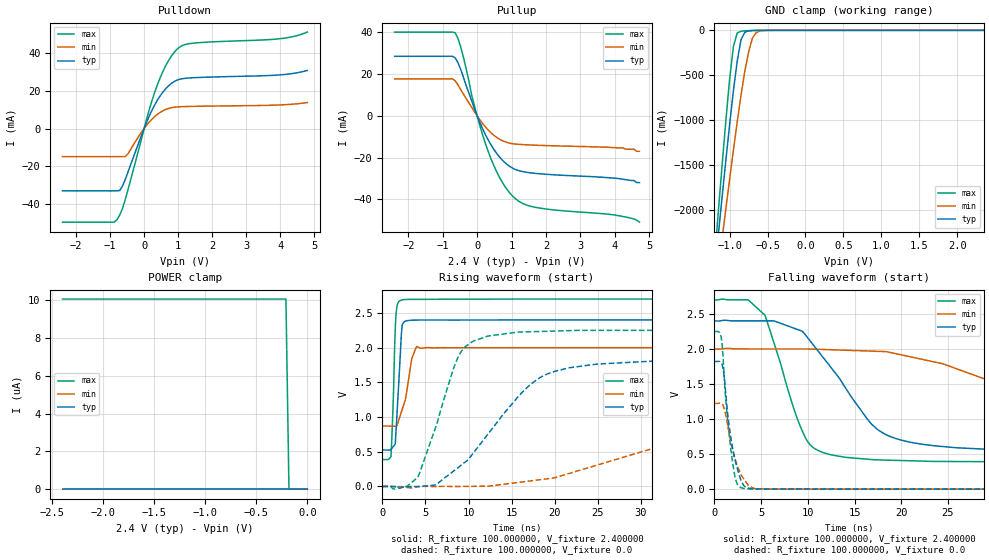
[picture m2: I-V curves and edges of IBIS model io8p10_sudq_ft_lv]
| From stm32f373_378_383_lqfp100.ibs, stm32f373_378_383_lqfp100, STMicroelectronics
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|   Model io8p10_sudq_ft_lv
[Model]  io8p10_sudq_ft_lv
Model_type I/O
Polarity   Non-Inverting
Enable   Active-Low
Vinl =   0.720000V
Vinh =   1.680000V
Vmeas =  1.200000V
Cref =   50.000000pF
Rref =   100.000000M
Vref =   0.0V
C_comp   1.970100pF   1.887900pF   2.069400pF
[Temperature Range]   25.000000   0.125000k   -40.000000
[Pullup Reference]   2.400000V   2.000000V   2.700000V
[Pulldown Reference]   0.0V   0.0V   0.0V
[POWER Clamp Reference]   2.400000V   2.000000V   2.700000V
[GND Clamp Reference]   0.0V   0.0V   0.0V
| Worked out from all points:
|   slope of the pulldown table from 0 to 0.36 V, typ, clamps not added: 25.5 ohm
|   slope of the pullup table from 0 to 0.36 V, typ, clamps not added: 28.4 ohm
|   GND clamp passes 1 mA (typ) near -0.64 V on its own axis
|   rising waveform, R_fixture 100.000000, V_fixture 2.400000: 20-80 % time 501ps typ, 1.06ns min, 336ps max; typ from 0.525 V to 2.4 V
|   rising waveform, R_fixture 100.000000, V_fixture 0.0: 20-80 % time 7.32ns typ, 21.7ns min, 3.52ns max; typ from 0 V to 1.82 V
|   falling waveform, R_fixture 100.000000, V_fixture 2.400000: 20-80 % time 6.27ns typ, 18.5ns min, 3.33ns max; typ from 2.4 V to 0.525 V
|   falling waveform, R_fixture 100.000000, V_fixture 0.0: 20-80 % time 1.16ns typ, 1.4ns min, 914ps max; typ from 1.82 V to 0 V
[Pulldown]
|Voltage   I(typ)   I(min)   I(max)
-2.4V     -33.16mA   -14.98mA   -49.86mA
-880mV    -33.16mA   -14.98mA   -49.86mA
-800mV    -33.16mA   -14.98mA   -48.55mA
-640mV    -30.75mA   -14.98mA   -42.76mA
-480mV    -23.43mA   -13.57mA   -32.92mA
80mV      3.651mA    1.905mA    5.506mA
400mV     15.37mA    7.665mA    23.73mA
720mV     22.75mA    10.69mA    36.23mA
1.04V     26.18mA    11.57mA    43.27mA
1.52V     27.09mA    11.81mA    45.55mA
4V        28.55mA    12.55mA    47.81mA
4.8V      30.9mA     13.81mA    51.31mA
[Pullup]
|Voltage   I(typ)   I(min)   I(max)
-2.4V     28.57mA    17.75mA    40.17mA
-720mV    28.57mA    17.75mA    40.17mA
-640mV    27.85mA    16.83mA    39.88mA
-480mV    22.38mA    12.65mA    33.22mA
-80mV     3.427mA    2.066mA    4.957mA
160mV     -6.219mA   -3.715mA   -9.137mA
320mV     -11.51mA   -6.781mA   -16.98mA
720mV     -21mA      -11.8mA    -31.54mA
1.12V     -25.77mA   -13.54mA   -39.82mA
1.76V     -27.69mA   -14.12mA   -44.07mA
4V        -29.9mA    -15.2mA    -47.5mA
4.72V     -32mA      -17mA      -51mA
[GND_clamp]
|Voltage   I(typ)   I(min)   I(max)
-2.4V     -9.788A    -9.782A    -9.734A
-1.2V     -2.718A    -3.02A     -2.568A
-1.15V    -2.29A     -2.675A    -2.036A
-1.1V     -1.868A    -2.333A    -1.515A
-1.05V    -1.454A    -1.995A    -1.012A
-950mV    -674.5mA   -1.337A    -180.5mA
-900mV    -345.2mA   -1.023A    -29.72mA
-850mV    -106.4mA   -726mA     -10.13mA
-750mV    -6.396mA   -244mA     -4.026mA
-700mV    -2.558mA   -88.61mA   -2.329mA
-600mV    -416uA     -7.739mA   -368uA
2.35V     0A         0A         0A
[POWER_clamp]
|Voltage   I(typ)   I(min)   I(max)
-2.4V     0A         0A         10.06uA
-210mV    0A         0A         10.06uA
-180mV    0A         0A         0A
0V        0A         0A         0A
[Ramp]
| variable   typ   min   max
dV/dt_r  1.09308/7.31082n   0.73308/21.71145n   1.34964/3.51759n
dV/dt_f  1.12481/6.26349n   0.67631/18.49686n   1.38754/3.32485n
R_load = 100.000000
[Rising Waveform]
R_fixture= 100.000000
V_fixture= 2.400000
V_fixture_min= 2.000000
V_fixture_max= 2.700000
|time   V(typ)   V(min)   V(max)
0s        525.2mV    870.3mV    387.4mV
1.001ns   533.2mV    868.7mV    426.9mV
1.301ns   579.1mV    867.1mV    1.388V
1.502ns   617.1mV    866.5mV    2.304V
1.702ns   1.054V     877mV      2.604V
2.202ns   2.189V     1.072V     2.684V
2.603ns   2.379V     1.227V     2.693V
3.403ns   2.395V     1.838V     2.696V
4.004ns   2.397V     2.017V     2.696V
49.85ns   2.4V       2V         2.7V
[Rising Waveform]
R_fixture= 100.000000
V_fixture= 0.0
V_fixture_min= 0.0
V_fixture_max= 0.0
|time   V(typ)   V(min)   V(max)
0s        1.81nV     16.19nV    1.388nV
2.803ns   -3.281mV   -14.07mV   -1.578mV
4.204ns   -1.834mV   -2.504mV   153.3mV
8.809ns   274.6mV    -1.375mV   1.87V
12.21ns   748.9mV    4.656mV    2.166V
18.02ns   1.547V     92.84mV    2.232V
24.82ns   1.763V     304.5mV    2.249V
40.24ns   1.817V     861.6mV    2.249V
51.85ns   1.822V     1.107V     2.249V
99.7ns    1.822V     1.223V     2.249V
[Falling Waveform]
R_fixture= 100.000000
V_fixture= 2.400000
V_fixture_min= 2.000000
V_fixture_max= 2.700000
|time   V(typ)   V(min)   V(max)
0s        2.4V       2V         2.7V
3.604ns   2.401V     2V         2.703V
5.405ns   2.402V     2V         2.482V
9.81ns    2.189V     2V         715.2mV
14.01ns   1.448V     1.982V     453.6mV
18.22ns   786.7mV    1.963V     414.6mV
25.83ns   591.3mV    1.722V     393.9mV
36.04ns   545.2mV    1.277V     387.5mV
53.05ns   528.1mV    942.3mV    387.4mV
99.7ns    525.2mV    870.3mV    387.4mV
[Falling Waveform]
R_fixture= 100.000000
V_fixture= 0.0
V_fixture_min= 0.0
V_fixture_max= 0.0
|time   V(typ)   V(min)   V(max)
0s        1.822V     1.223V     2.249V
700.7ps   1.802V     1.222V     2.18V
800.8ps   1.785V     1.215V     2.098V
1.001ns   1.656V     1.165V     1.707V
1.401ns   1.093V     924.2mV    997.1mV
1.902ns   616.8mV    592mV      421.8mV
2.302ns   368.5mV    388.7mV    122.4mV
2.903ns   107.4mV    191.2mV    17.72mV
4.705ns   2.748mV    4.47mV     1.93mV
49.85ns   1.81nV     16.19nV    1.388nV
